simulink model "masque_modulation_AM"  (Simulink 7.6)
settings: Solver=ode15s  StartTime=0.0  StopTime=3e-3  RelTol=1e-3
InitFcn:
  | Xm=1;
  | fm=1e3;
  | 
  | % amplitude et fréquence de la porteuse
  | Xp=5;
  | fp=50e3;
  | 
  | % taux de modulation
  | m=0.5;
StopFcn:
  | close all, clc
  | load modulation_AM.mat
  | plot(x(1,:),x(2,:),x(1,:),x(3,:))
  | title('Signal modulé et modulant - Modulation d''amplitude')
  | xlabel('temps')
  | grid
libraries: fl_lib x17, nesl_utility x2, elec_lib x1

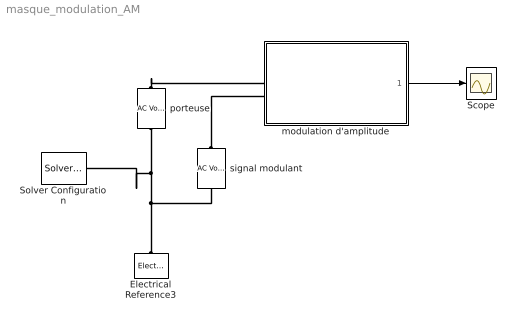
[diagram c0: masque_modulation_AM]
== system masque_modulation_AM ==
  Electrical Reference3 : fl_lib/Electrical/Electrical Elements/Electrical Reference  DialogController=NetworkEngine.DynNeDlgSource  SystemSampleTime=-1  i_Log=off  LocalVarNames=|i  LocalVarDescs=|i  LocalVarLogging=0
  Scope : Scope
  Solver Configuration : nesl_utility/Solver Configuration  DialogController=NetworkEngine.DynNeUtilDlgSource  SystemSampleTime=-1  PhysicalDomain=network_engine_domain  LeftPortType=input  RightPortType=generic  SubClassName=solver  Accelerate=off  Profile=off  ResidualTolerance=1e-9  MaxNonlinIter=3  MaxModeIter=2  DoFixedCost=off  UseLocalSampling=off  DoDC=off  LinearAlgebra=Sparse  LocalSolverSampleTime=.001  LocalSolverChoice=NE_BACKWARD_EULER_ADVANCER  UseLocalSolver=off
  modulation d'amplitude : Subsystem
  porteuse : fl_lib/Electrical/Electrical Sources/AC Voltage Source  DialogController=NetworkEngine.DynNeDlgSource  SystemSampleTime=-1  amp=Xp V  shift=0 rad  omega=fp Hz  i_Log=off  v_Log=off  LocalVarNames=|i|v  LocalVarDescs=|i|v  LocalVarLogging=[0 0]
  signal modulant : fl_lib/Electrical/Electrical Sources/AC Voltage Source  DialogController=NetworkEngine.DynNeDlgSource  SystemSampleTime=-1  amp=Xm V  shift=0 rad  omega=fm Hz  i_Log=off  v_Log=off  LocalVarNames=|i|v  LocalVarDescs=|i|v  LocalVarLogging=[0 0]
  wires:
  modulation d'amplitude/1(signal modulé) -> Scope/1
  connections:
  porteuse/LConn1 -- modulation d'amplitude/LConn1
  signal modulant/LConn1 -- modulation d'amplitude/LConn2
  porteuse/RConn1 -- Electrical Reference3/LConn1 -- signal modulant/RConn1 -- Solver Configuration/RConn1

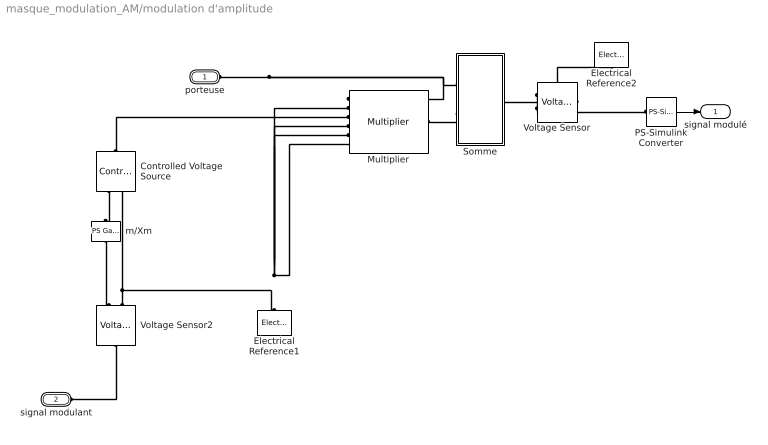
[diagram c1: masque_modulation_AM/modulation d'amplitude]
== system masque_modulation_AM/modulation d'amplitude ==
  Controlled Voltage Source : fl_lib/Electrical/Electrical Sources/Controlled Voltage Source  DialogController=NetworkEngine.DynNeDlgSource  SystemSampleTime=-1  i_Log=off  v_Log=off  LocalVarNames=|i|v  LocalVarDescs=|i|v  LocalVarLogging=[0 0]
  Electrical Reference1 : fl_lib/Electrical/Electrical Elements/Electrical Reference  DialogController=NetworkEngine.DynNeDlgSource  SystemSampleTime=-1  i_Log=off  LocalVarNames=|i  LocalVarDescs=|i  LocalVarLogging=0
  Electrical Reference2 : fl_lib/Electrical/Electrical Elements/Electrical Reference  DialogController=NetworkEngine.DynNeDlgSource  SystemSampleTime=-1  i_Log=off  LocalVarNames=|i  LocalVarDescs=|i  LocalVarLogging=0
  Multiplier : elec_lib/Integrated Circuits/Multiplier  DialogController=NetworkEngine.DynNeDlgSource  SystemSampleTime=-1  K=1 V  A=1  Rin=1e+7 Ohm  Vdiff=15 V  Rout=0.1 Ohm  Vmin=-15 V  Vmax=15 V  Vdotmax=20 V/us  f=1 MHz  V0=0 V  LocalVarLogging=[]
  PS-Simulink Converter : nesl_utility/PS-Simulink Converter  DialogController=NetworkEngine.DynNeUtilDlgSource  SystemSampleTime=-1  PhysicalDomain=network_engine_domain  LeftPortType=input  RightPortType=output  SubClassName=ps_output  Unit=1  AffineConversion=off
  Somme : Subsystem
  Voltage Sensor : fl_lib/Electrical/Electrical Sensors/Voltage Sensor  DialogController=NetworkEngine.DynNeDlgSource  SystemSampleTime=-1  i1_Log=off  v1_Log=off  LocalVarNames=|i1|v1  LocalVarDescs=|i1|v1  LocalVarLogging=[0 0]
  Voltage Sensor2 : fl_lib/Electrical/Electrical Sensors/Voltage Sensor  DialogController=NetworkEngine.DynNeDlgSource  SystemSampleTime=-1  i1_Log=off  v1_Log=off  LocalVarNames=|i1|v1  LocalVarDescs=|i1|v1  LocalVarLogging=[0 0]
  m/Xm : fl_lib/Physical Signals/Functions/PS Gain  DialogController=NetworkEngine.DynNeDlgSource  SystemSampleTime=-1  gain=m/Xm  LocalVarLogging=[]
  porteuse : PMIOPort  Port=1  Side=Left
  signal modulant : PMIOPort  Port=2  Side=Left
  signal modulé : Outport
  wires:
  PS-Simulink Converter/1 -> signal modulé/1
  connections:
  Voltage Sensor2/LConn1 -- signal modulant/RConn1
  m/Xm/LConn1 -- Voltage Sensor2/RConn1
  Somme/RConn1 -- Voltage Sensor/LConn1
  Voltage Sensor/RConn1 -- PS-Simulink Converter/LConn1
  Somme/LConn2 -- Multiplier/RConn1
  Somme/LConn1 -- porteuse/RConn1 -- Multiplier/LConn1
  Voltage Sensor/RConn2 -- Electrical Reference2/LConn1
  Voltage Sensor2/RConn2 -- Multiplier/LConn6 -- Multiplier/LConn5 -- Multiplier/LConn2 -- Multiplier/LConn4 -- Electrical Reference1/LConn1 -- Controlled Voltage Source/RConn2
  Controlled Voltage Source/RConn1 -- m/Xm/RConn1
  Controlled Voltage Source/LConn1 -- Multiplier/LConn3

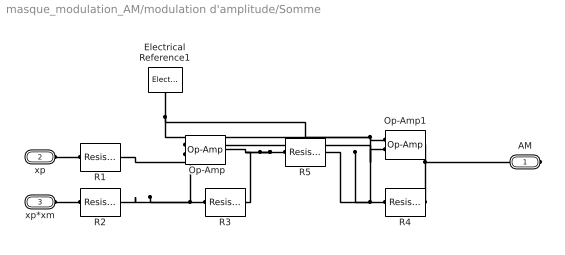
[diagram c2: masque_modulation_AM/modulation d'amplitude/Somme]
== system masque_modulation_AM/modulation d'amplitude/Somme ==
  Electrical Reference1 : fl_lib/Electrical/Electrical Elements/Electrical Reference  DialogController=NetworkEngine.DynNeDlgSource  SystemSampleTime=-1  i_Log=off  LocalVarNames=|i  LocalVarDescs=|i  LocalVarLogging=0
  Op-Amp : fl_lib/Electrical/Electrical Elements/Op-Amp  DialogController=NetworkEngine.DynNeDlgSource  SystemSampleTime=-1  i1_Log=off  v1_Log=off  outI_Log=off  LocalVarNames=|i1|v1|outI  LocalVarDescs=|i1|v1|outI  LocalVarLogging=[0 0 0]
  Op-Amp1 : fl_lib/Electrical/Electrical Elements/Op-Amp  DialogController=NetworkEngine.DynNeDlgSource  SystemSampleTime=-1  i1_Log=off  v1_Log=off  outI_Log=off  LocalVarNames=|i1|v1|outI  LocalVarDescs=|i1|v1|outI  LocalVarLogging=[0 0 0]
  R1 : fl_lib/Electrical/Electrical Elements/Resistor  DialogController=NetworkEngine.DynNeDlgSource  SystemSampleTime=-1  R=1 Ohm  i_Log=off  v_Log=off  LocalVarNames=|i|v  LocalVarDescs=|i|v  LocalVarLogging=[0 0]
  R2 : fl_lib/Electrical/Electrical Elements/Resistor  DialogController=NetworkEngine.DynNeDlgSource  SystemSampleTime=-1  R=1 Ohm  i_Log=off  v_Log=off  LocalVarNames=|i|v  LocalVarDescs=|i|v  LocalVarLogging=[0 0]
  R3 : fl_lib/Electrical/Electrical Elements/Resistor  DialogController=NetworkEngine.DynNeDlgSource  SystemSampleTime=-1  R=1 Ohm  i_Log=off  v_Log=off  LocalVarNames=|i|v  LocalVarDescs=|i|v  LocalVarLogging=[0 0]
  R4 : fl_lib/Electrical/Electrical Elements/Resistor  DialogController=NetworkEngine.DynNeDlgSource  SystemSampleTime=-1  R=1 kOhm  i_Log=off  v_Log=off  LocalVarNames=|i|v  LocalVarDescs=|i|v  LocalVarLogging=[0 0]
  R5 : fl_lib/Electrical/Electrical Elements/Resistor  DialogController=NetworkEngine.DynNeDlgSource  SystemSampleTime=-1  R=1 kOhm  i_Log=off  v_Log=off  LocalVarNames=|i|v  LocalVarDescs=|i|v  LocalVarLogging=[0 0]
  AM : PMIOPort  Port=1  Side=Right
  xp : PMIOPort  Port=2  Side=Left
  xp*xm : PMIOPort  Port=3  Side=Left
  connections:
  R4/LConn1 -- Op-Amp1/LConn2 -- R5/RConn1
  R4/RConn1 -- AM/RConn1 -- Op-Amp1/RConn1
  xp*xm/RConn1 -- R2/LConn1
  xp/RConn1 -- R1/LConn1
  R5/LConn1 -- Op-Amp/RConn1 -- R3/RConn1
  R3/LConn1 -- R2/RConn1 -- R1/RConn1 -- Op-Amp/LConn2
  Op-Amp1/LConn1 -- Op-Amp/LConn1 -- Electrical Reference1/LConn1
